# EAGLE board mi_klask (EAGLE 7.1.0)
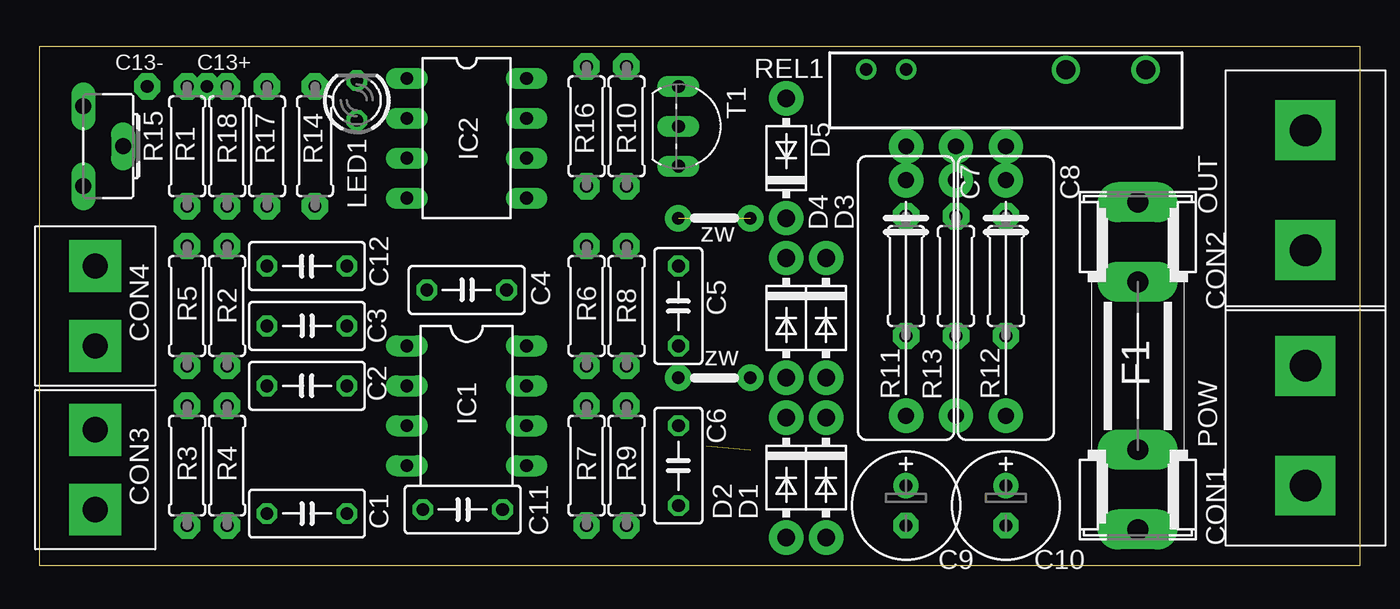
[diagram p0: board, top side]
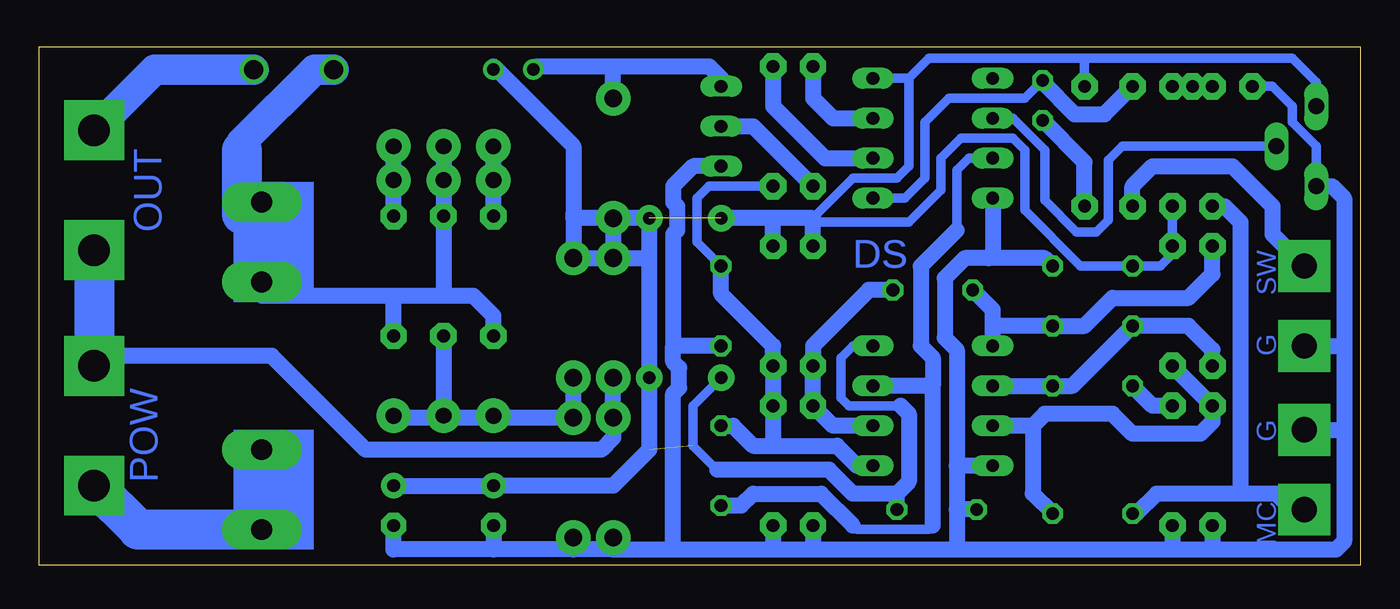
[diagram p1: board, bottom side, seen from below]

Size 84 x 33 mm. Coordinates in mm from the lower left corner, seen from the top.
Outline: 0,33 0,0 84,0 84,33 0,33
Copper layers (1*16): Top 0.035mm / dielectric 1.5mm / Bottom 0.035mm
Design rules "default": minimum track width 10mil, minimum drill 24mil, track to track 8mil, track to pad 8mil, pad to pad 8mil, via to via 8mil, smd to smd 8mil, copper to edge 40mil, drill to drill 8mil, minimum pad ring 10mil, minimum via ring 8mil, stop-mask expansion 4mil, vias tented up to drill 0mil, thermal gap 10mil

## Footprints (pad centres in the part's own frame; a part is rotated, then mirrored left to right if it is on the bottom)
C050-030X075 = drill 0.813 octagon: 1 -2.54,0; 2 2.54,0
C150-064X183 = drill 1.016 octagon: 1 -7.493,0; 2 7.493,0
E2,5-7 = drill 0.813 pad 1.6: + -1.27,0 | drill 0.813 pad 1.6 octagon: - 1.27,0
ARK2/750 = drill 2 pad 3.81 square: 1 -3.81,0; 2 3.81,0
ARK2/500 = drill 1.6 pad 3.302 square: 1 -2.54,0; 2 2.54,0
DO41-10 = drill 1.118 pad 2.184: A 3.81,0; C -3.81,0
SHK20L = drill 1.321 pad 2.54 long: 1A -10.414,0; 1B -5.334,0; 2A 10.414,0; 2B 5.334,0
DIL08 = drill 0.813 pad 1.27 long: 1 -3.81,-3.81; 2 -1.27,-3.81; 3 1.27,-3.81; 4 3.81,-3.81; 5 3.81,3.81; 6 1.27,3.81; 7 -1.27,3.81; 8 -3.81,3.81
DIL08' = drill 0.813 long: 1 -3.81,-3.81; 2 -1.27,-3.81; 3 1.27,-3.81; 4 3.81,-3.81; 5 3.81,3.81; 6 1.27,3.81; 7 -1.27,3.81; 8 -3.81,3.81
LED3MM = drill 0.813 octagon: A -1.27,0; K 1.27,0
0207/7 = drill 0.813 pad 1.676 octagon: 1 -3.81,0; 2 3.81,0
CA6H = drill 1.016 long: A -2.54,0; E 2.54,0; S 0,2.54
PA-CLI-SOCKET = drill 0.8: 1 -8.89,1.32; 2 -6.35,1.32 | drill 1.2: COM 8.89,1.32; NO 3.81,1.32
TO92-EBC = drill 0.813 long: B 0,-1.27; C -2.54,-1.27; E 2.54,-1.27

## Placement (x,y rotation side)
C1  [C050-030X075]  17.02,3.28 0 top
C2  [C050-030X075]  17.02,11.41 180 top
C3  [C050-030X075]  17.02,15.22 0 top
C4  [C050-030X075]  27.18,17.51 0 top
C5  [C050-030X075]  40.64,16.49 270 top
C6  [C050-030X075]  40.64,6.33 90 top
C7  [C150-064X183]  55.12,17 270 top
C8  [C150-064X183]  61.47,17 270 top
C9  [E2,5-7]  55.12,3.79 270 top
C10  [E2,5-7]  61.47,3.79 270 top
C11  [C050-030X075]  26.92,3.54 0 top
C12  [C050-030X075]  17.02,19.03 180 top
CON1  POW  [ARK2/750]  80.52,8.87 90 top
CON2  OUT  [ARK2/750]  80.52,23.86 90 top
CON3  MIC  [ARK2/500]  3.56,6.08 90 top
CON4  SW  [ARK2/500]  3.56,16.49 90 top
D1  5V1  [DO41-10]  50.04,5.57 270 top
D2  5V1  [DO41-10]  47.5,5.57 270 top
D3  4007  [DO41-10]  50.04,15.73 270 top
D4  4007  [DO41-10]  47.5,15.73 270 top
D5  4007  [DO41-10]  47.5,25.89 90 top
F1  [SHK20L]  69.85,12.68 90 top
IC1  TL062P  [DIL08]  27.18,10.14 270 top
IC2  ATTINY25  [DIL08']  27.18,27.16 270 top
LED1  [LED3MM]  20.19,29.57 90 top
R1  [0207/7]  9.4,26.65 90 top
R2  [0207/7]  11.94,16.49 90 top
R3  [0207/7]  9.4,6.33 90 top
R4  [0207/7]  11.94,6.33 90 top
R5  [0207/7]  9.4,16.49 270 top
R6  [0207/7]  34.8,16.49 270 top
R7  [0207/7]  34.8,6.33 90 top
R8  [0207/7]  37.34,16.49 90 top
R9  [0207/7]  37.34,6.33 270 top
R10  [0207/7]  37.34,27.92 90 top
R11  [0207/7]  55.12,18.39 270 top
R12  [0207/7]  61.47,18.39 270 top
R13  [0207/7]  58.29,18.39 90 top
R14  [0207/7]  17.53,26.65 270 top
R15  [CA6H]  2.79,26.65 270 top
R16  [0207/7]  34.8,27.92 90 top
R17  [0207/7]  14.48,26.65 270 top
R18  [0207/7]  11.94,26.65 90 top
REL1  [PA-CLI-SOCKET]  61.47,30.21 0 top
T1  BC548  [TO92-EBC]  41.91,27.92 270 top

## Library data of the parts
C1-C12 R1-R14 R16-R18 = rcl
CON1-CON4 = dimmer
D1-D5 = diode
F1 = fuse; OC_FARNELL: unknown; OC_NEWARK: unknown
IC1 = linear
IC2 = avr-7
LED1 = led
R15 = pot
REL1 = relay; OC_FARNELL: unknown; OC_NEWARK: unknown
T1 = transistor-npn

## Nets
AC1: F1.2A R11.2 R12.2 R13.2 REL1.NO
LED: IC2.5 LED1.K R17.1
LVL: IC2.6 R10.2
N$1: C1.1 CON3.1 R1.1
N$2: C7.2 C8.2 D1.C D3.A R13.1
N$3: C1.2 IC1.3 R2.1 R3.2
N$4: R16.1 T1.B
N$5: C4.2 IC1.6 R6.2 R7.2
N$6: C3.2 C4.1 IC1.1 R5.1
N$7: C2.2 R4.2
N$8: CON4.2 R17.2
N$9: C2.1 C3.1 IC1.2 R5.2
N$10: C5.1 C6.2 IC1.5 R8.1 R9.1 R10.1
N$11: C7.1 R11.1
N$12: C8.1 R12.1
N$13: LED1.A R14.2
N$14: CON1.2 CON2.1 D2.C D4.A
N$15: CON1.1 F1.1A
N$16: CON2.2 REL1.COM
N$17: R1.2 R18.2
N$21: C5.2 C9.- C10.- C11.1 C12.1 CON3.2 CON4.1 D1.A D2.A IC1.4 IC2.4 R3.1 R4.1 R7.1 R9.2 R15.E T1.E
REG: IC2.2 R15.S
REL: IC2.7 R16.2
RELS: D5.A REL1.1 T1.C
SIG: C6.1 IC1.7 IC2.3
VDD: C9.+ C10.+ C11.2 C12.2 D3.C D4.C D5.C IC1.8 IC2.8 R2.2 R6.1 R8.2 R14.1 R15.A R18.1 REL1.2

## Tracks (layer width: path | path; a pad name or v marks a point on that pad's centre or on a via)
AC1  (via drill 1 pad 2.18)
  Bottom 1.016: R11.2 55.12,15.85 56.39,17.12 58.29,17.12 | 58.29,17.12 61.47,17.12 | 61.47,17.12 69.85,17.12 F1.2A | R12.2 61.47,17.12 | 58.29,17.12 R13.2 v58.29,24.49 v58.29,26.65
  Bottom 1.93: REL1.NO 66.5,31.53 71.12,26.9 71.12,26.4
  Bottom 2.54: 71.12,26.4 71.12,22.33 F1.2A
LED
  Bottom 0.61: IC2.5 28.96,23.35 27.69,24.62 27.69,28.17 26.16,29.7 21.34,29.7 LED1.K
  Bottom 1.016: LED1.K 20.19,30.71 18.16,28.68 16.26,28.68 R17.1
LVL
  Bottom 1.016: R10.2 37.34,29.19 34.04,25.89 IC2.6
N$1
  Bottom 1.016: CON3.1 4.32,3.54 5.33,4.55 7.62,4.55 | 7.62,4.55 12.95,4.55 14.22,3.28 C1.1 | R1.1 8.64,22.84 7.62,21.82 7.62,4.55
N$2
  Bottom 1.016: D3.A D1.C 54.99,9.38 | 54.99,9.38 58.55,9.38 | 58.55,9.38 61.34,9.38 C8.2 | C7.2 54.99,9.38 | R13.1 58.29,9.63 58.55,9.38
N$3
  Bottom 1.016: 20.83,8.87 20.83,4.55 C1.2 | 20.83,8.87 20.07,9.63 15.75,9.63 14.48,8.36 10.16,8.36 9.4,9.12 R3.2 R2.1 | 20.83,8.87 IC1.3
N$4
  Bottom 1.016: T1.B 38.61,27.92 R16.1
N$5
  Bottom 1.016: C4.2 31.24,17.51 34.8,13.95 R6.2 R7.2 33.53,8.87 IC1.6
N$6
  Bottom 1.016: IC1.1 23.37,15.47 | 23.37,15.47 23.37,16.24 C4.1 | 23.37,15.47 23.11,15.22 C3.2 17.53,15.22 15.75,17 10.92,17 9.4,18.52 R5.1
N$7
  Bottom 1.016: R4.2 13.21,10.14 C2.2
N$8
  Bottom 1.016: R17.2 14.48,24.11 13.21,25.38 8.13,25.38 5.59,22.84 5.59,21.06 CON4.2
N$9
  Bottom 1.016: IC1.2 C2.1 18.29,11.41 C3.1 10.92,15.22 9.4,13.7 R5.2
N$10
  Bottom 0.61: R10.1 41.4,24.11 42.16,23.35 42.16,20.55 C5.1
  Bottom 1.016: C5.1 40.64,17.25 37.34,13.95 R8.1 R9.1 37.34,7.85 37.59,7.6 | IC1.5 32,6.33 33.27,7.6 37.59,7.6 | C6.2 39.88,8.87 38.61,7.6 37.59,7.6
N$11  (via drill 1 pad 2.18)
  Bottom 1.016: R11.1 C7.1 v55.12,26.65
N$12  (via drill 1 pad 2.18)
  Bottom 1.016: R12.1 C8.1 v61.47,26.65
N$13
  Bottom 1.016: R14.2 17.53,25.63 LED1.A
N$14
  Bottom 1.016: 80.52,13.31 69.22,13.31 63.25,7.35 48.26,7.35 47.5,8.11 D2.C D4.A
  Bottom 2.54: CON2.1 80.52,13.31 CON1.2
N$15
  Bottom 2.54: CON1.1 77.72,2.27 F1.1A
N$16
  Bottom 1.93: REL1.COM 76.66,31.53 CON2.2
N$17
  Bottom 1.016: R1.2 R18.2
N$18  (via drill 0.8 pad 1.68)
  other vias: 10.67,30.46
N$19  (via drill 1 pad 2.18)
  other vias: 55.12,24.49
N$20  (via drill 1 pad 2.18)
  other vias: 61.47,24.49
N$21  (via drill 0.8 pad 1.68)
  Bottom 0.61: v6.86,30.46 5.59,30.46 4.32,29.19 4.32,28.17 2.79,26.65 R15.E
  Bottom 1.016: D1.A 50.04,1 | 50.04,1 55.12,1 | 55.12,1 61.47,1 C10.- | C9.- 55.12,1 | D2.A 47.5,1 | 47.5,1 50.04,1 | T1.E 42.42,25.38 43.69,24.11 43.69,23.09 43.43,22.84 43.43,21.32 43.69,21.06 43.69,13.95 | 47.5,1 43.69,1 | 43.69,1 37.34,1 | 37.34,1 34.8,1 | 34.8,1 25.65,1 | 25.65,1 11.94,1 | 11.94,1 9.4,1 | 9.4,1 1.52,1 1.02,1.5 1.02,8.62 | C5.2 43.69,13.95 | R9.2 37.34,1 | R7.1 34.8,1 | 43.69,1 43.69,10.9 43.31,11.28 43.31,12.55 43.69,12.93 43.69,13.95 | 25.65,6.33 25.65,13.7 26.42,14.46 26.42,18.27 25.15,19.54 23.62,19.54 | 25.65,6.33 25.65,3.54 | 25.65,3.54 25.65,1 | IC1.4 25.65,6.33 | C11.1 25.65,3.54 | 1.02,13.95 1.02,23.35 1.78,24.11 R15.E | 1.02,13.95 1.02,8.62 | C12.1 20.07,19.54 23.62,19.54 | IC2.4 23.37,19.79 23.62,19.54 | R3.1 9.4,1 | R4.1 11.94,1 | CON3.2 1.02,8.62 | CON4.1 1.02,13.95
N$22  (via drill 1 pad 2.18)
  other vias: 55.12,9.51
N$23  (via drill 1 pad 2.18)
  other vias: 61.47,9.51
REG
  Bottom 0.61: IC2.2 22.1,28.43 20.07,26.4 20.07,23.22 18.03,21.19 16.76,21.19 16,21.95 16,25.76 15.11,26.65 R15.S
REL
  Bottom 1.016: R16.2 34.8,29.7 33.53,28.43 IC2.7
RELS
  Bottom 1.016: REL1.1 52.32,31.73 47.5,31.73 | 47.5,31.73 41.4,31.73 40.64,30.97 T1.C | D5.A 47.5,31.73
S$1  (via drill 1 pad 2.18)
  other vias: 58.29,9.51
SIG
  Bottom 0.61: 32.26,2.52 32,2.27 27.43,2.27 27.18,2.52 | IC2.3 24.89,25.89 25.65,25.13 25.65,21.32
  Bottom 1.016: 27.18,11.41 27.18,13.19 27.94,13.95 27.94,19.03 25.65,21.32 | 27.18,11.41 IC1.7 | C6.1 39.37,3.79 38.61,4.55 34.29,4.55 32.26,2.52 | 27.18,2.52 27.18,11.41
VDD  (via drill 0.8 pad 1.68)  (2 unrouted)
  Bottom 0.61: 29.21,10.14 32.51,10.14 33.02,10.65 33.02,13.19 32.26,13.95 IC1.8 | 40.89,6.08 42.42,7.6 42.42,10.14 v40.64,11.92 | 28.7,30.97 28.7,25.38 29.46,24.62 32.26,24.62 34.8,22.08 | IC2.8 28.7,30.97 | 17.53,32.24 4.32,32.24 2.79,30.71 R15.A | 17.53,32.24 27.43,32.24 28.7,30.97 | R14.1 17.53,32.24 | 34.8,21.82 28.7,21.82 26.67,23.86 26.67,25.89 25.4,27.16 22.1,27.16 21.34,26.4 21.34,22.59 17.78,19.03 C12.2 12.7,19.03 11.94,19.79 R2.2 R18.1
  Bottom 1.016: C10.+ C9.+ 47.5,5.06 45.21,7.35 v45.21,11.92 45.21,19.54 | D4.C D3.C 50.04,22.08 49.78,22.08 | 29.21,10.14 28.7,9.63 28.7,5.31 29.46,4.55 | 29.46,4.55 32.26,4.55 33.78,6.08 40.89,6.08 | 45.21,19.54 v45.21,22.08 D5.C | D4.C 45.21,19.54 | D5.C 49.78,22.08 | D5.C D4.C | REL1.2 55.12,31.73 50.04,26.65 50.04,22.33 49.78,22.08 | R6.1 34.8,21.82 34.8,22.08 37.34,22.08 | 37.34,22.08 v40.64,22.08 | R8.2 37.34,22.08 | C11.2 29.46,4.55
(copper drawn outside any net)
  shapes: Bottom area x2

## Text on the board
Bottom: OUT | SW | DS | DS | G | POW | G | MC
tPlace: C13- | C13+ | OUT | zw | zw | POW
